TYPE STR_EX260_SEC :
STRUCT
	A:USINT;
	B:USINT;
	C:USINT;
	D:USINT;
	(*
	Out_Bit0	:	BOOL	;
	Out_Bit1	:	BOOL	;
	Out_Bit2	:	BOOL	;
	Out_Bit3	:	BOOL	;
	Out_Bit4	:	BOOL	;
	Out_Bit5	:	BOOL	;
	Out_Bit6	:	BOOL	;
	Out_Bit7	:	BOOL	;
	Out_Bit8	:	BOOL	;
	Out_Bit9	:	BOOL	;
	Out_Bit10	:	BOOL	;
	Out_Bit11	:	BOOL	;
	Out_Bit12	:	BOOL	;
	Out_Bit13	:	BOOL	;
	Out_Bit14	:	BOOL	;
	Out_Bit15	:	BOOL	;
	Out_Bit16	:	BOOL	;
	Out_Bit17	:	BOOL	;
	Out_Bit18	:	BOOL	;
	Out_Bit19	:	BOOL	;
	Out_Bit20	:	BOOL	;
	Out_Bit21	:	BOOL	;
	Out_Bit22	:	BOOL	;
	Out_Bit23	:	BOOL	;
	Out_Bit24	:	BOOL	;
	Out_Bit25	:	BOOL	;
	Out_Bit26	:	BOOL	;
	Out_Bit27	:	BOOL	;
	Out_Bit28	:	BOOL	;
	Out_Bit29	:	BOOL	;
	Out_Bit30	:	BOOL	;
	Out_Bit31	:	BOOL	;
	*)

END_STRUCT
END_TYPE
